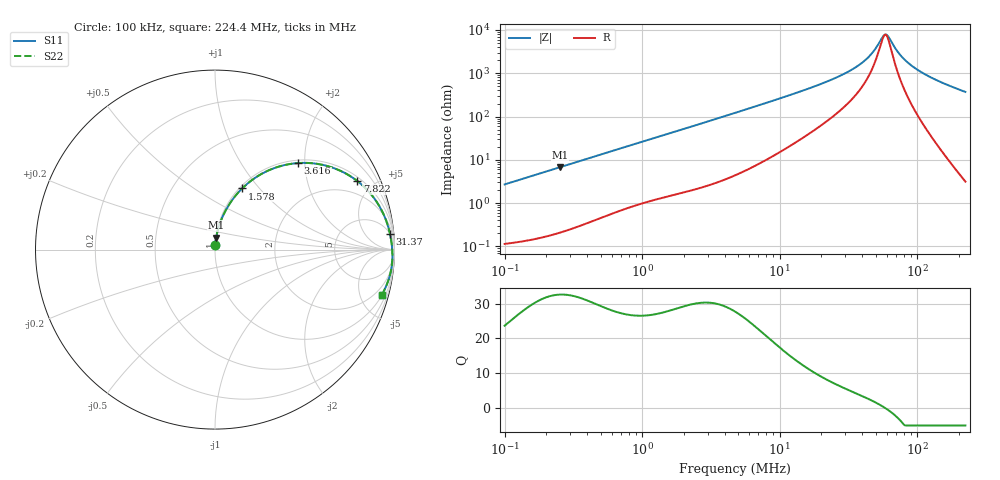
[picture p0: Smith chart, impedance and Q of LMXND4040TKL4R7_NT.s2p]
! LMXND4040TKL4R7_NT  S-PARAMETER MODEL  ( Standard Model )
! Model Generated by TAIYO YUDEN Corporation (https://www.yuden.co.jp/en/)
! Version 1.0
! TAIYO YUDEN Control No. 20250409
! Copyright(c) 2025 TAIYO YUDEN CO.,LTD. All Rights Reserved.
! Product Description (link to TY-COMPAS)
! https://ds.yuden.co.jp/TYCOMPAS/or/detail?pn=LMXND4040TKL4R7MNT&u=M
! Products Name : Inductors
! Characteristics :
!  Inductance : 4.7 [uH] , SRF(min) : 35 [MHz] , DC Resistance(max) : 0.084 [Ohm]
!  Rated Current : Saturation  2000 [mA] , Temp Rise  2300 [mA] (40 [degC])
!  Case Size : 4.0 x 4.0 / 0.157 x 0.157 [mm/inch] , Thickness : 1.8 / 0.071 [mm/inch]
!  (Conditions: Temperature = 25 [degC] , DC Bias Current = 0 [A])
! External Node Assignments :
!  1  o---GGG---o  2
! GND o---------o GND
! Frequency Range : 0.1MHz  -  224.402193MHz  [ 402 STEP ]
# MHz S RI R 50
! Freq[MHz].  S11 Real  S11 Imag  S21 Real  S21 Imag  S12 Real  S12 Imag  S22 Real  S22 Imag
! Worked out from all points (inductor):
!   401 points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, 100 kHz to 224.4 MHz, reference 50 ohm
!   read as one part in series: L = 4.29 uH near 103.9 kHz
!   highest Q = 32.6 at 252.4 kHz (marker M1), where L = 4.27 uH
!   self-resonance near 58.16 MHz
!   S11 on the Smith chart (normalised r, x): 100 kHz: 1.00, +0.05; 1.578 MHz: 1.03, +0.81; 3.616 MHz: 1.06, +1.85; 7.822 MHz: 1.19, +4.04; 31.37 MHz: 5, +21; 224.4 MHz: 1.06, -7.41
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0.1  0.00187 0.0269  0.9981 -0.0269  0.9981 -0.0269  0.00187 0.0269
0.25242  0.00661 0.0671  0.9934 -0.0671  0.9934 -0.0671  0.00661 0.0671
0.364164  0.0124 0.0958  0.9876 -0.0958  0.9876 -0.0958  0.0124 0.0958
0.77272  0.0463 0.1923  0.9537 -0.1923  0.9537 -0.1923  0.0463 0.1923
1.326154  0.1143 0.3004  0.8857 -0.3004  0.8857 -0.3004  0.1143 0.3004
1.577583  0.1509 0.3406  0.8491 -0.3406  0.8491 -0.3406  0.1509 0.3406
2.320297  0.2684 0.4267  0.7316 -0.4267  0.7316 -0.4267  0.2684 0.4267
3.615993  0.4625 0.4821  0.5375 -0.4821  0.5375 -0.4821  0.4625 0.4821
4.737111  0.5922 0.4737  0.4078 -0.4737  0.4078 -0.4737  0.5922 0.4737
7.822225  0.7922 0.3826  0.2078 -0.3826  0.2078 -0.3826  0.7922 0.3826
17.25085  0.9407 0.1935  0.0593 -0.1935  0.0593 -0.1935  0.9407 0.1935
31.37005  0.975 0.0876  0.025 -0.0876  0.025 -0.0876  0.975 0.0876
38.04441  0.9804 0.0594  0.0196 -0.0594  0.0196 -0.0594  0.9804 0.0594
44.39268  0.9836 0.038  0.0164 -0.038  0.0164 -0.038  0.9836 0.038
48.88766  0.9852 0.0248  0.0148 -0.0248  0.0148 -0.0248  0.9852 0.0248
57.04529  0.9872 0.0038  0.0128 -0.0038  0.0128 -0.0038  0.9872 0.0038
59.28911  0.9875 -0.00151  0.0125 0.00151  0.0125 0.00151  0.9875 -0.00151
62.8214  0.988 -0.00954  0.012 0.00954  0.012 0.00954  0.988 -0.00954
76.18743  0.9885 -0.0373  0.0115 0.0373  0.0115 0.0373  0.9885 -0.0373
96.03159  0.9867 -0.0734  0.0133 0.0734  0.0133 0.0734  0.9867 -0.0734
138.5441  0.9751 -0.1402  0.0249 0.1402  0.0249 0.1402  0.9751 -0.1402
224.4022  0.9302 -0.2506  0.0698 0.2506  0.0698 0.2506  0.9302 -0.2506
